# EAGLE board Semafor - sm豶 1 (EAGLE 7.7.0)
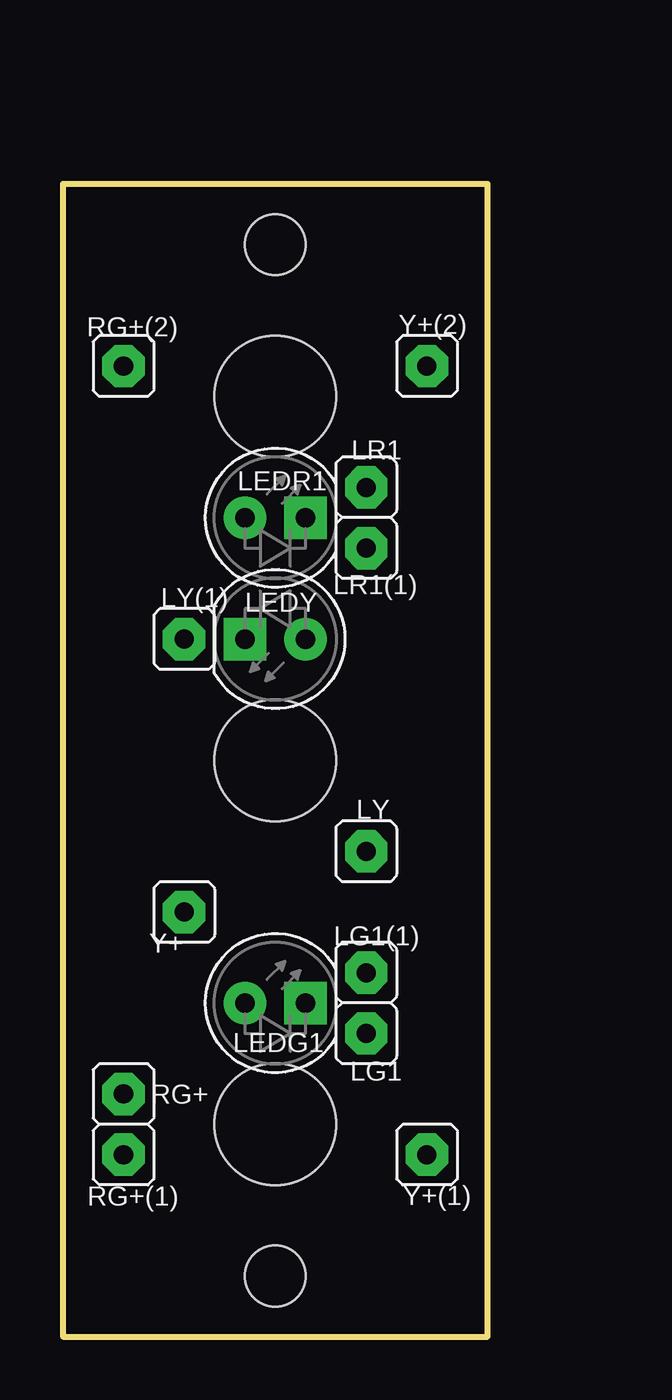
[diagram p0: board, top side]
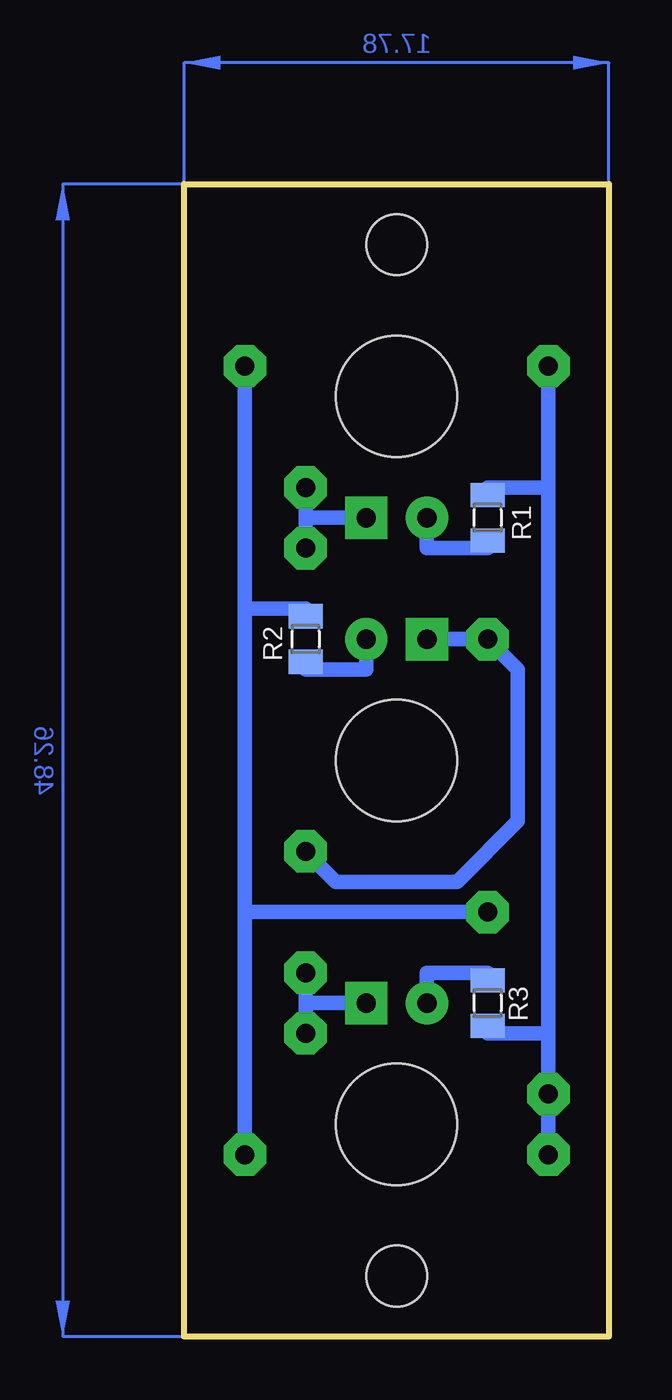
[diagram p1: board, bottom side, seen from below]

Size 17.78 x 48.26 mm. Coordinates in mm from the lower left corner, seen from the top.
Outline: 0,0 17.78,0 17.78,48.26 0,48.26 0,0
Copper layers (1*16): Top 0.035mm / dielectric 1.5mm / Bottom 0.035mm
Design rules "default": minimum track width 10mil, minimum drill 24mil, track to track 8mil, track to pad 8mil, pad to pad 8mil, via to via 8mil, smd to smd 8mil, copper to edge 40mil, drill to drill 8mil, minimum pad ring 10mil, minimum via ring 8mil, stop-mask expansion 4mil, vias tented up to drill 0mil, thermal gap 10mil
Holes 5.08 mm at 8.89,8.89 8.89,24.13 8.89,39.37
Holes 2.54 mm at 8.89,2.54 8.89,45.72

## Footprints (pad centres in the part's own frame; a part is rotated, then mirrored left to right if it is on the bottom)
LED_5 = drill 0.813 pad 1.778: A -1.27,0 | drill 0.813 pad 1.778 square: K 1.27,0
S1G1_JUM = drill 0.8 pad 1.778 octagon: 1 0,0
0805 = smd 1.016 x 1.422: 1 -0.953,0; 2 0.953,0

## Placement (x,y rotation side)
LEDG1  [LED_5]  8.89,13.97 0 top
LEDR1  [LED_5]  8.89,34.29 0 top
LEDY  [LED_5]  8.89,29.21 180 top
LG1  [S1G1_JUM]  12.7,12.7 0 top
LG1(1)  [S1G1_JUM]  12.7,15.24 0 top
LR1  [S1G1_JUM]  12.7,35.56 0 top
LR1(1)  [S1G1_JUM]  12.7,33.02 0 top
LY  [S1G1_JUM]  12.7,20.32 0 top
LY(1)  [S1G1_JUM]  5.08,29.21 0 top
R1  680R  [0805]  5.08,34.29 270 bottom
R2  680R  [0805]  12.7,29.21 270 bottom
R3  680R  [0805]  5.08,13.97 90 bottom
RG+  [S1G1_JUM]  2.54,10.16 0 top
RG+(1)  [S1G1_JUM]  2.54,7.62 0 top
RG+(2)  [S1G1_JUM]  2.54,40.64 0 top
Y+  [S1G1_JUM]  5.08,17.78 0 top
Y+(1)  [S1G1_JUM]  15.24,7.62 0 top
Y+(2)  [S1G1_JUM]  15.24,40.64 0 top

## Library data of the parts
LEDG1 LEDR1 LEDY R1-R3 = 1pomocná
LG1 LG1(1) LR1 LR1(1) LY LY(1) RG+ RG+(1) RG+(2) Y+ Y+(1) Y+(2) = #PaJa_konektory

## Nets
N$1: LEDR1.A R1.2
N$2: R1.1 R3.1 RG+(1).1 RG+(2).1 RG+.1
N$3: LEDR1.K LR1(1).1 LR1.1
N$4: LEDY.A R2.2
N$5: R2.1 Y+(1).1 Y+(2).1 Y+.1
N$6: LEDY.K LY(1).1 LY.1
N$7: LEDG1.A R3.2
N$9: LEDG1.K LG1(1).1 LG1.1

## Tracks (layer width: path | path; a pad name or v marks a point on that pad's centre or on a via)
N$1
  Bottom 0.61: LEDR1.A 7.62,33.02 5.08,33.02 R1.2
N$2
  Bottom 0.61: 2.54,12.7 RG+.1 RG+(1).1 | 2.54,12.7 2.54,35.56 | 2.54,35.56 RG+(2).1 | R1.1 5.08,35.56 2.54,35.56 | R3.1 5.08,12.7 2.54,12.7
N$3
  Bottom 0.61: LEDR1.K 12.7,34.29 | 12.7,34.29 LR1.1 | 12.7,34.29 LR1(1).1
N$4
  Bottom 0.61: LEDY.A 10.16,27.94 12.7,27.94 R2.2
N$5
  Bottom 0.61: 15.24,30.48 Y+(2).1 | R2.1 12.7,30.48 15.24,30.48 | 15.24,30.48 15.24,17.78 | 15.24,17.78 Y+(1).1 | Y+.1 15.24,17.78
N$6
  Bottom 0.61: LEDY.K LY(1).1 3.81,27.94 3.81,21.59 6.35,19.05 11.43,19.05 LY.1
N$7
  Bottom 0.61: LEDG1.A 7.62,15.24 5.08,15.24 R3.2
N$9
  Bottom 0.61: LEDG1.K 12.7,13.97 | 12.7,13.97 LG1(1).1 | 12.7,13.97 LG1.1
(copper drawn outside any net)
  shapes: Bottom area x2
